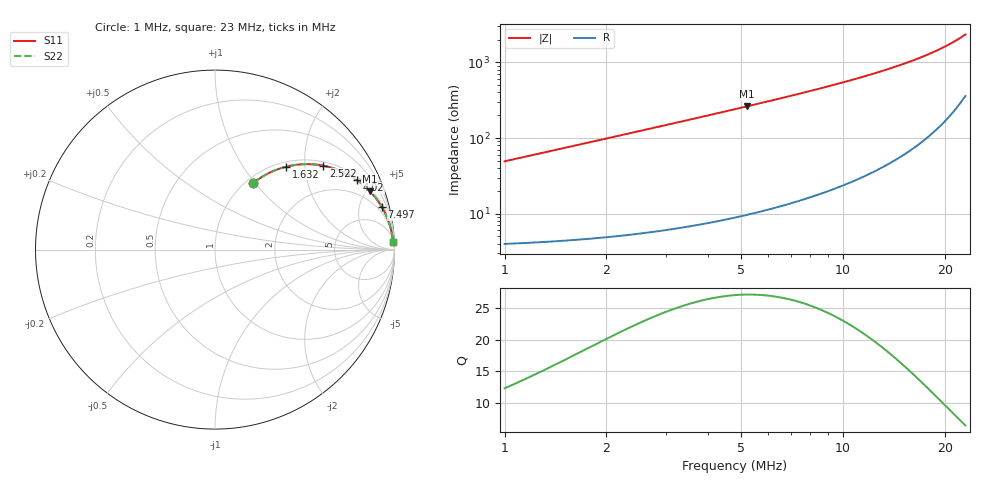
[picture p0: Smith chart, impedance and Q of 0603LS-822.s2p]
# MHz S MA R 50
!Freq  MagS11  AngS11  MagS21  AngS21  MagS12  AngS12  MagS22  AngS22
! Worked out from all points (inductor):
!   801 points, 1 MHz to 23 MHz, reference 50 ohm
!   read as one part in series: L = 7.81 uH near 1.016 MHz
!   highest Q = 27.2 at 5.187 MHz (marker M1), where L = 8.01 uH
!   S11 on the Smith chart (normalised r, x): 1 MHz: 1.08, +0.98; 1.632 MHz: 1.09, +1.60; 2.522 MHz: 1.11, +2.49; 4.02 MHz: 1.15, +4.00; 7.497 MHz: 1.30, +7.78; 23 MHz: 8, +46
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1  0.4281 60.1  0.8698 -25.3  0.8698 -25.3  0.4281 60.1
1.156059  0.4797 57.3  0.8435 -28.6  0.8435 -28.6  0.4797 57.3
1.300303  0.5234 54.7  0.8183 -31.5  0.8183 -31.5  0.5234 54.7
1.632187  0.6097 49.3  0.7591 -37.5  0.7591 -37.5  0.6097 49.3
2.032783  0.6908 43.6  0.6899 -43.6  0.6899 -43.6  0.6908 43.6
2.521795  0.7633 37.8  0.6133 -49.7  0.6133 -49.7  0.7633 37.8
2.858767  0.8007 34.5  0.5666 -53.1  0.5666 -53.1  0.8007 34.5
3.215464  0.8321 31.5  0.5224 -56.2  0.5224 -56.2  0.8321 31.5
3.602519  0.8589 28.7  0.48 -59.1  0.48 -59.1  0.8589 28.7
4.020377  0.8815 26.1  0.4401 -61.7  0.4401 -61.7  0.8815 26.1
4.684368  0.908 22.7  0.3868 -65.1  0.3868 -65.1  0.908 22.7
5.186891  0.9226 20.7  0.3532 -67.2  0.3532 -67.2  0.9226 20.7
6.236036  0.9439 17.3  0.2969 -70.6  0.2969 -70.6  0.9439 17.3
7.497391  0.9596 14.3  0.2467 -73.5  0.2467 -73.5  0.9596 14.3
8.334287  0.9667 12.7  0.2204 -75.0  0.2204 -75.0  0.9667 12.7
10.0594  0.9763 10.3  0.1782 -77.2  0.1782 -77.2  0.9763 10.3
12.04679  0.9828 8.2  0.1426 -79.0  0.1426 -79.0  0.9828 8.2
15.726  0.9889 5.6  0.09705 -80.7  0.09705 -80.7  0.9889 5.6
19.35677  0.9915 3.8  0.06603 -80.7  0.06603 -80.7  0.9915 3.8
21.0999  0.9922 3.1  0.05404 -80.1  0.05404 -80.1  0.9922 3.1
22.64223  0.9925 2.5  0.04454 -79.1  0.04454 -79.1  0.9925 2.5
23  0.9926 2.4  0.04247 -78.7  0.04247 -78.7  0.9926 2.4
